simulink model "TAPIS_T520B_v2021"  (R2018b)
settings: Solver=ode23t  StartTime=0.0  StopTime=10  RelTol=1e-3  EnableMultiTasking=on
libraries: fl_lib x13, nesl_utility x5, elec_lib x1

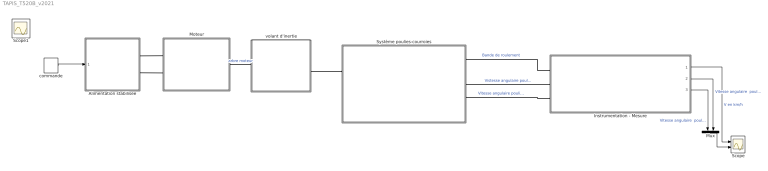
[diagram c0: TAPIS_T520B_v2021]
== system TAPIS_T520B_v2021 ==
  Alimentation stabilisee : Subsystem
  Instrumentation - Mesure : Subsystem
  Moteur : Subsystem  mask{R=1, L=1.2e-5, Kv=0.5, J=0.001, Cs=0.076936, Cv=0.000159}
      mask prompts: R "Résistance interne R en Ohms"; L "Inductance de l'induit L en Henrys"; Kv "Constante de vitesse Kv en V/(rad/s)"; J "Moment d'inertie du Moteur J en Kg.m²"; Cs "Couple de frottements secs Cs en N.m"; Cv "Couple de frottements visqueux Cv en N.m/(rad/s)"
  Mux : Mux  Inputs=2
  Scope : Scope  NumInputPorts=2
  Système poulies-courroies : Subsystem  mask{rapportreduction=1, rayonrouleau=0.0195}
      mask prompts: rapportreduction "Rapport de réduction du système poulies-courroie"; rayonrouleau "Rayon du rouleau entrainant r en m"
  commande : DiscretePulseGenerator  PulseType=Time based  Amplitude=180  Period=10  PulseWidth=50  PhaseDelay=2
  volant d'inertie : Subsystem  mask{inertie=0.001}
      mask prompts: inertie "Inertie en kg.m²"
  Scope1 : Scope
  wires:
  commande/1 -> Alimentation stabilisee/1(In1)
  Mux/1 -> Scope/2
  Instrumentation - Mesure/3(Vitesse angulaire poulie menante en rad/s) -> Mux/1  "Vitesse angulaire  poulie menée"
  Instrumentation - Mesure/1(Vitesse linéaire en km/h) -> Scope/1  "V en km/h"
  Instrumentation - Mesure/2(Vitesse angulaire poulie menée en rad/s) -> Mux/2  "Vitesse angulaire  poulie menante"
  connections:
  Moteur/LConn1 -- Alimentation stabilisee/RConn1
  volant d'inertie/LConn1 -- Moteur/RConn1  "arbre moteur"
  Système poulies-courroies/RConn4 -- Instrumentation - Mesure/LConn3  "Vitesse angulaire poulie menée"
  Système poulies-courroies/RConn3 -- Instrumentation - Mesure/LConn2  "Vistesse angulaire poulie menante"
  Système poulies-courroies/RConn1 -- Instrumentation - Mesure/LConn1  "Bande de roulement"
  volant d'inertie/RConn1 -- Système poulies-courroies/LConn1
  Alimentation stabilisee/RConn2 -- Moteur/LConn2

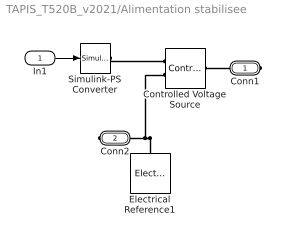
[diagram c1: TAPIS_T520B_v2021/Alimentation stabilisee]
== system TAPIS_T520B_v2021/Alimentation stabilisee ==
  In1 : Inport
  Controlled Voltage Source : fl_lib/Electrical/Electrical Sources/Controlled Voltage Source
  Electrical Reference1 : fl_lib/Electrical/Electrical Elements/Electrical Reference
  Simulink-PS Converter : nesl_utility/Simulink-PS Converter  PhysicalDomain=network_engine_domain  SubClassName=ps_input  LeftPortType=input  RightPortType=output  PseudoPeriodic=off  Frequencies=[]  NoiseDistribution=none  NoiseParameters=[]  Unit=1  AffineConversion=off  FilteringAndDerivatives=zero  SimscapeFilterOrder=1  InputFilterTimeConstant=.001  UdotUserProvided=0
  Conn1 : PMIOPort  Side=Right
  Conn2 : PMIOPort  Port=2  Side=Right
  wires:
  In1/1 -> Simulink-PS Converter/1
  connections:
  Simulink-PS Converter/RConn1 -- Controlled Voltage Source/RConn1
  Conn2/RConn1 -- Electrical Reference1/LConn1 -- Controlled Voltage Source/RConn2
  Conn1/RConn1 -- Controlled Voltage Source/LConn1

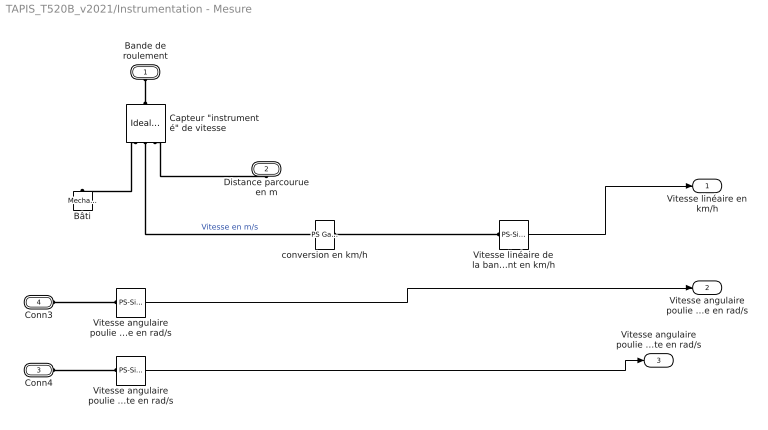
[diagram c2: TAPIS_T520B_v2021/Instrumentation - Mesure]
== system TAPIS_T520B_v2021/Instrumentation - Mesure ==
  Bâti : fl_lib/Mechanical/Translational Elements/Mechanical Translational Reference
  "Capteur \"instrumenté\" de vitesse" : fl_lib/Mechanical/Mechanical Sensors/Ideal Translational Motion Sensor  offset=0 m
  Vitesse angulaire poulie menante en rad/s : nesl_utility/PS-Simulink Converter  PhysicalDomain=network_engine_domain  SubClassName=ps_output  LeftPortType=input  RightPortType=output  PseudoPeriodic=off  Frequencies=[]  Unit=rad/s  AffineConversion=off
  Vitesse angulaire poulie menée en rad/s : nesl_utility/PS-Simulink Converter  PhysicalDomain=network_engine_domain  SubClassName=ps_output  LeftPortType=input  RightPortType=output  PseudoPeriodic=off  Frequencies=[]  Unit=rad/s  AffineConversion=off
  Vitesse linéaire de la bande de roulement en km/h : nesl_utility/PS-Simulink Converter  PhysicalDomain=network_engine_domain  SubClassName=ps_output  LeftPortType=input  RightPortType=output  PseudoPeriodic=off  Frequencies=[]  Unit=1  AffineConversion=off
  conversion en km/h : fl_lib/Physical Signals/Functions/PS Gain  gain=3.6
  Bande de roulement : PMIOPort  Side=Left
  Distance parcourue en m : PMIOPort  Port=2  Side=Right
  Conn4 : PMIOPort  Port=3  Side=Left
  Conn3 : PMIOPort  Port=4  Side=Left
  Vitesse linéaire en km/h : Outport
  Vitesse angulaire poulie menée en rad/s : Outport  Port=2
  Vitesse angulaire poulie menante en rad/s : Outport  Port=3
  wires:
  Vitesse linéaire de la bande de roulement en km/h/1 -> Vitesse linéaire en km/h/1
  Vitesse angulaire poulie menée en rad/s/1 -> Vitesse angulaire poulie menée en rad/s/1
  Vitesse angulaire poulie menante en rad/s/1 -> Vitesse angulaire poulie menante en rad/s/1
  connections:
  Bâti/LConn1 -- "Capteur \"instrumenté\" de vitesse"/RConn1
  "Capteur \"instrumenté\" de vitesse"/RConn2 -- conversion en km/h/LConn1  "Vitesse en m/s"
  conversion en km/h/RConn1 -- Vitesse linéaire de la bande de roulement en km/h/LConn1
  Bande de roulement/RConn1 -- "Capteur \"instrumenté\" de vitesse"/LConn1
  Distance parcourue en m/RConn1 -- "Capteur \"instrumenté\" de vitesse"/RConn3
  Conn3/RConn1 -- Vitesse angulaire poulie menée en rad/s/LConn1
  Conn4/RConn1 -- Vitesse angulaire poulie menante en rad/s/LConn1

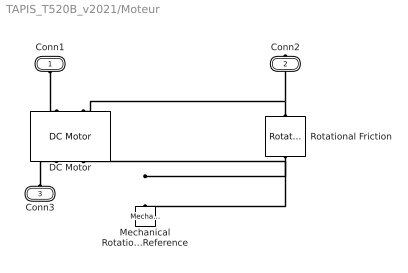
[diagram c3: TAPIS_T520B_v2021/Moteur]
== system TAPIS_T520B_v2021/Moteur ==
  DC Motor : elec_lib/Actuators & Drivers/Rotational Actuators/DC Motor  parameterization=1  Ra=R Ohm  La=L H  emf_or_torque=1  Kv=Kv V/(rad/s)  Ki=6.876e-4 N*m/A  T_stall=2.4e-4 N*m  w_max=1.91e+4 rpm  w_rated=1.5e+4 rpm  P_rated=0.08 W  V_rated=1.5 V  J=0.000971 kg*m^2  lam_param=1  lam=0 N*m/(rad/s)  i_noload=0 A  V_i_noload=1.5 V  speed0=0 rpm  alpha=3.93e-3 1/K  Tmeas=25 degC  thermal_mass=100 J/K  initial_temperature=25 degC
  Mechanical Rotational Reference : fl_lib/Mechanical/Rotational Elements/Mechanical Rotational Reference
  Rotational Friction : fl_lib/Mechanical/Rotational Elements/Rotational Friction  brkwy_trq=Cs*1.25 N*m  brkwy_vel=0.60653 rad/s  Col_trq=Cs N*m  visc_coef=Cv N*m/(rad/s)  w_specify=off  w_priority=None  w=0 rad/s  w_nominal_specify=off  w_nominal_unit=rad/s  w_nominal_value=1  t_specify=off  t_priority=None  t=0 N*m  t_nominal_specify=off  t_nominal_unit=N*m  t_nominal_value=1
  Conn1 : PMIOPort  Side=Left
  Conn2 : PMIOPort  Port=2  Side=Right
  Conn3 : PMIOPort  Port=3  Side=Left
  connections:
  Conn1/RConn1 -- DC Motor/LConn1
  Rotational Friction/LConn1 -- DC Motor/LConn2 -- Conn2/RConn1
  Conn3/RConn1 -- DC Motor/RConn1
  Rotational Friction/RConn1 -- DC Motor/RConn2 -- Mechanical Rotational Reference/LConn1

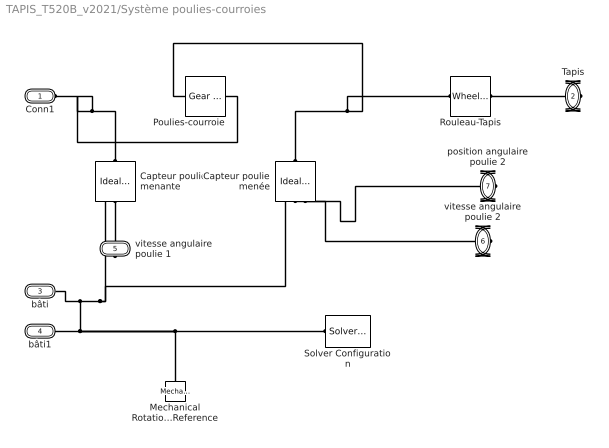
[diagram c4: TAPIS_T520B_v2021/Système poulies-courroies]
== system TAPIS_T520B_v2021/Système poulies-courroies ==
  Capteur poulie menée : fl_lib/Mechanical/Mechanical Sensors/Ideal Rotational Motion Sensor  offset=0 rad
  Capteur poulie menante : fl_lib/Mechanical/Mechanical Sensors/Ideal Rotational Motion Sensor  offset=0 rad
  Mechanical Rotational Reference : fl_lib/Mechanical/Rotational Elements/Mechanical Rotational Reference
  Poulies-courroie : fl_lib/Mechanical/Mechanisms/Gear Box  ratio=rapportreduction  t_in_specify=off  t_in_priority=None  t_in=0 N*m  t_in_nominal_specify=off  t_in_nominal_unit=N*m  t_in_nominal_value=1  t_out_specify=off  t_out_priority=None  t_out=0 N*m  t_out_nominal_specify=off  t_out_nominal_unit=N*m  t_out_nominal_value=1
  Rouleau-Tapis : fl_lib/Mechanical/Mechanisms/Wheel and Axle  R=rayonrouleau m  or=1  t_specify=off  t_priority=None  t=0 N*m  t_nominal_specify=off  t_nominal_unit=N*m  t_nominal_value=1  f_specify=off  f_priority=None  f=0 N  f_nominal_specify=off  f_nominal_unit=N  f_nominal_value=1
  Solver Configuration : nesl_utility/Solver Configuration  PhysicalDomain=network_engine_domain  SubClassName=solver  LeftPortType=input  RightPortType=generic  Tones=[]  Harmonics=[]  SimulateNoise=off  Profile=off  UseLocalSampling=off  EnableSwitchedLinearOptims=on  FrequencyDomain=off  UseCCode=off  RelTol=0.001  AbsTol=1e-06  MinStep=1e-09  ToWorkspace=off  RevertToSquareIcSolve=off  NumHomotopyIterations=100  PhasorMode=off  PhasorModeNumHarmonics=1  DoDC=on  ResidualTolerance=1e-9  UseLocalSolver=off  LocalSolverChoice=NE_BACKWARD_EULER_ADVANCER  LocalSolverSampleTime=.001  DoFixedCost=off  MaxNonlinIter=3  MaxModeIter=2  LinearAlgebra=Sparse  EquationFormulation=NE_TIME_EF  DelaysMemoryBudget=1024  AutomaticFiltering=on  FilteringTimeConstant=0.001  PartitionStorageMethod=AS_NEEDED  PartitionMemoryBudget=1024
  Conn1 : PMIOPort  Side=Left
  Tapis : PMIOPort  Port=2  Side=Right
  bâti : PMIOPort  Port=3  Side=Left
  bâti1 : PMIOPort  Port=4  Side=Right
  vitesse angulaire poulie 1 : PMIOPort  Port=5  Side=Right
  vitesse angulaire poulie 2 : PMIOPort  Port=6  Side=Right
  position angulaire poulie 2 : PMIOPort  Port=7  Side=Right
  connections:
  Capteur poulie menante/LConn1 -- Poulies-courroie/RConn1 -- Conn1/RConn1
  Capteur poulie menée/LConn1 -- Poulies-courroie/LConn1 -- Rouleau-Tapis/LConn1
  vitesse angulaire poulie 1/RConn1 -- Capteur poulie menante/RConn2
  Mechanical Rotational Reference/LConn1 -- Solver Configuration/RConn1 -- bâti/RConn1 -- Capteur poulie menante/RConn1 -- Capteur poulie menée/RConn1 -- bâti1/RConn1
  Tapis/RConn1 -- Rouleau-Tapis/RConn1
  vitesse angulaire poulie 2/RConn1 -- Capteur poulie menée/RConn2
  position angulaire poulie 2/RConn1 -- Capteur poulie menée/RConn3

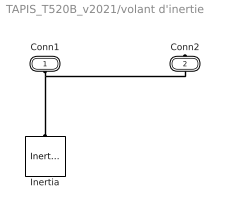
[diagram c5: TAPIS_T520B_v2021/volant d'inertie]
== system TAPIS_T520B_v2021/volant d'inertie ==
  Inertia : fl_lib/Mechanical/Rotational Elements/Inertia  inertia=inertie kg*m^2  w_specify=on  w_priority=High  w=0 rad/s  w_nominal_specify=off  w_nominal_unit=rad/s  w_nominal_value=1  t_specify=off  t_priority=None  t=0 N*m  t_nominal_specify=off  t_nominal_unit=N*m  t_nominal_value=1
  Conn1 : PMIOPort  Side=Left
  Conn2 : PMIOPort  Port=2  Side=Right
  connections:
  Conn1/RConn1 -- Conn2/RConn1 -- Inertia/LConn1
